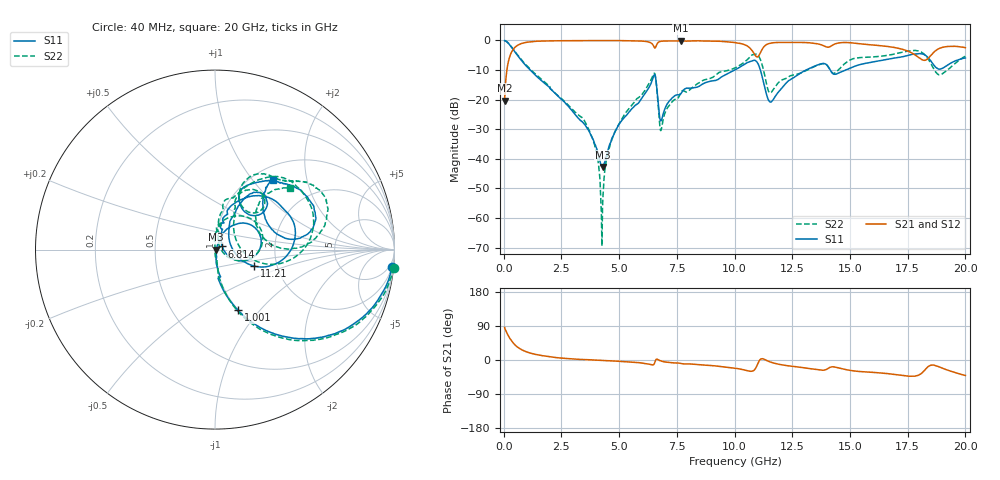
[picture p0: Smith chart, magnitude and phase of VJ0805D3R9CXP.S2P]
! VJ0805D3R9CXP
! DATE 10/29/2021  11:48
! CAPACITORS MOUNTED IN SERIES ON 25 MIL THICK MICROSTRIP SUBSTRATE
# GHz  S  MA  R  50.00
!  FREQ  S11M  S11A  S21M  S21A  S12M  S12A  S22M  S22A
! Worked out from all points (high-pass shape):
!   1601 points, 40 MHz to 20 GHz, reference 50 ohm
!   highest |S21| = -0.03 dB at 7.675 GHz (marker M1); lowest = -20.3 dB at 40 MHz (marker M2)
!   |S21| within 3 dB of the highest: 411.5 MHz to 10.72 GHz (10.31 GHz wide, 185 % of centre); 11.19 GHz to 17.3 GHz (6.101 GHz wide, 42.8 % of centre)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
!   lowest |S11| = -42.7 dB at 4.294 GHz (marker M3), VSWR 1.01, Z = 50.7 - j0.0264 ohm
!   |S11| at or under -10 dB: 1.142 GHz to 9.997 GHz (8.855 GHz wide, 159 % of centre); 11.12 GHz to 13.09 GHz (1.972 GHz wide, 16.3 % of centre); 14.15 GHz to 14.81 GHz (664.5 MHz wide, 4.59 % of centre)
!   |S22| runs from -69.5 to 0.0 dB; largest |S21 - S12| = 0.0063
!   S11 on the Smith chart (normalised r, x): 40 MHz: 2, -20; 1.001 GHz: 0.99, -0.77; 6.814 GHz: 1.08, +0.04; 11.21 GHz: 1.52, -0.30; 20 GHz: 1.22, +1.27
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0.04  0.9918 -5.6  0.09655 85.9  0.09435 84.0  0.9997 -5.8
0.326925  0.7805 -38.3  0.6187 51.7  0.6196 51.6  0.791 -38.5
1.000575  0.3615 -69.3  0.9327 21.2  0.9316 21.2  0.3742 -69.2
3.370825  0.04311 -77.6  0.9886 1.4  0.9882 1.4  0.0508 -79.0
3.95715  0.01731 -66.1  0.9941 -0.2  0.9942 -0.3  0.01586 -90.0
4.293975  0.007311 -2.0  0.9941 -1.2  0.9943 -1.3  0.002055 91.4
4.543475  0.01527 52.2  0.9946 -2.0  0.9946 -2.0  0.01392 89.3
5.192175  0.04841 62.0  0.9914 -4.2  0.9914 -4.3  0.05312 93.0
6.489575  0.247 32.6  0.8111 -12.6  0.8121 -12.6  0.2688 37.5
6.70165  0.08058 -25.0  0.9322 0.4  0.9326 0.3  0.07258 -28.7
6.813925  0.04389 23.9  0.9691 -2.7  0.9694 -2.8  0.03023 31.2
7.6747  0.126 75.8  0.9961 -9.0  0.9959 -9.2  0.1318 85.0
10.02  0.3187 61.5  0.9206 -21.5  0.9209 -21.7  0.3438 67.4
10.7186  0.4432 31.2  0.7065 -29.8  0.7076 -30.1  0.5531 46.3
11.20513  0.2372 -22.8  0.7179 3.5  0.718 3.1  0.3757 -11.8
11.55443  0.09072 18.9  0.8994 -5.4  0.8986 -5.5  0.1294 25.0
13.35083  0.3522 58.5  0.9058 -23.5  0.9049 -23.7  0.3456 65.7
16.68165  0.4842 52.5  0.7851 -36.4  0.7854 -36.6  0.5644 42.5
17.96657  0.5968 25.6  0.5187 -40.2  0.5189 -40.5  0.664 19.0
18.49053  0.459 7.5  0.5521 -13.9  0.5513 -14.2  0.4148 0.3
18.92715  0.3281 31.6  0.7489 -19.8  0.7489 -19.9  0.2667 28.3
20  0.5049 50.4  0.7523 -40.9  0.7532 -41.1  0.5412 39.4
